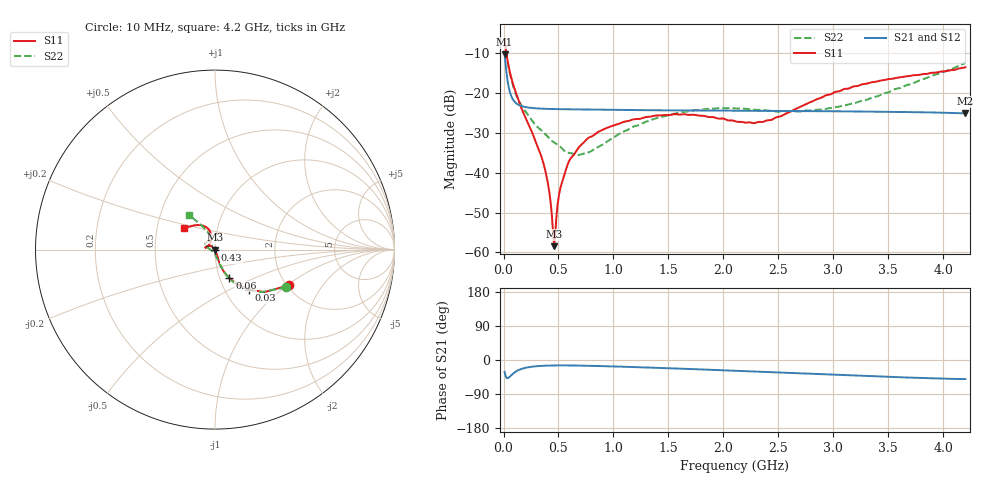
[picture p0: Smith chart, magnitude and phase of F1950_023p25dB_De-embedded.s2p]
! Integrated Device Technology
! Corporate Headquarters
! 6024 Silver Creek Valley Road
! San Jose, CA 95138  USA
! Phone:  1-408-284-8200
! Toll Free:  1-800-223-1366
! Webpage:  http://www.idt.com/
! Timing and RF Division
! 515 Groton Road, Suite 102
! Westford, MA 01886-6024
! Device:  F1950
! Description: 7-bit 0.25 dB Digital Step Attenuator
! Frequency:  150.0 -  4000.00 MHz
! Package:  4x4 mm Thin QFN Plastic Package: 24 pin
! Ports:  2 RF, 12 DC
!  Pin  1  = D0
!  Pin  2  = VDD
!  Pin  3  = Vmode
!  Pin  4  = GND
!  Pin  5  = RF1  =  Port 1
!  Pin  6  = GND
!  Pin  7  = GND
!  Pin  8  = GND
!  Pin  9  = GND
!  Pin 10  = GND
!  Pin 11  = GND
!  Pin 12  = GND
!  Pin 13  = GND
!  Pin 14  = RF2  =  Port 2
!  Pin 15  = GND
!  Pin 16  = LE
!  Pin 17  = CLK
!  Pin 18  = DATE
!  Pin 19  = D6
!  Pin 20  = D5
!  Pin 21  = D4
!  Pin 22  = D3
!  Pin 23  = D2
!  Pin 24  = D1
! State:  93
! Atten State:  23.25 dB
! Voltage:  +5.00 Volts
! Current:  Not Measured mA
! Data:  The device was measured on a the F195X evaluation board which has
!  individual transmission lines to the RF pins.  Data was collected
!  using a calibrated network analyzer.  The evaluation board was
!  de-embedded using a TRL calibration technique.
!  The reference plane is the edge of the package pin.
! Misc:  Board 2019
!  Action Tracker AT0250
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# GHz S dB R 50
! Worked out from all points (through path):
!   420 points, 10 MHz to 4.2 GHz, reference 50 ohm
!   highest |S21| = -10.24 dB at 10 MHz (marker M1); lowest = -25.1 dB at 4.2 GHz (marker M2)
!   group delay of S21, straight-line fit = 23.8 ps
!   lowest |S11| = -58.5 dB at 460 MHz (marker M3), VSWR 1.00, Z = 49.9 - j0.0633 ohm
!   |S11| at or under -10 dB: 26.59 MHz to end of sweep
!   |S22| runs from -35.6 to -6.9 dB; largest |S21 - S12| = 0.00012
!   S11 on the Smith chart (normalised r, x): 10 MHz: 2.06, -1.03; 30 MHz: 1.30, -0.63; 60 MHz: 1.11, -0.36; 430 MHz: 1.00, -0.01; 4.2 GHz: 0.69, +0.17
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0.01  -6.78 -25.7  -10.24 -31.1  -10.24 -31.1  -6.95 -28.0
0.03  -10.63 -49.5  -15.53 -47.8  -15.53 -47.8  -11.02 -51.6
0.06  -15.02 -62.9  -19.94 -43.2  -19.94 -43.2  -15.26 -64.2
0.1  -18.89 -69.8  -22.15 -33.0  -22.15 -33.0  -19.29 -69.4
0.15  -22.83 -71.8  -23.12 -25.0  -23.12 -25.1  -22.50 -73.5
0.35  -36.42 -68.3  -23.92 -15.4  -23.92 -15.4  -29.47 -83.5
0.4  -42.14 -71.3  -23.97 -14.8  -23.97 -14.8  -30.85 -85.3
0.43  -47.86 -81.4  -24.00 -14.5  -23.99 -14.6  -31.71 -88.2
0.45  -54.86 -103.2  -24.01 -14.4  -24.01 -14.4  -32.22 -91.5
0.46  -58.46 -147.9  -24.02 -14.4  -24.02 -14.4  -32.41 -93.1
0.48  -51.46 146.7  -24.03 -14.3  -24.03 -14.3  -32.73 -96.1
0.51  -44.77 137.7  -24.05 -14.3  -24.05 -14.3  -33.28 -99.0
0.57  -39.05 133.1  -24.07 -14.3  -24.07 -14.3  -34.86 -109.6
0.71  -32.93 137.0  -24.13 -14.8  -24.13 -14.9  -35.33 -138.9
1  -28.11 147.3  -24.22 -17.0  -24.22 -17.0  -31.15 178.5
1.41  -25.64 162.6  -24.33 -20.9  -24.32 -20.9  -26.16 160.0
1.73  -25.45 167.9  -24.37 -24.1  -24.37 -24.1  -24.32 151.7
2.11  -27.11 157.3  -24.44 -28.5  -24.44 -28.5  -23.88 141.8
2.43  -26.78 125.5  -24.48 -31.9  -24.48 -32.0  -24.44 130.9
2.81  -22.07 104.8  -24.54 -36.5  -24.54 -36.6  -24.40 115.4
3.51  -16.46 117.0  -24.69 -44.5  -24.69 -44.6  -19.71 112.6
4.2  -13.52 145.5  -25.10 -50.4  -25.09 -50.5  -12.45 126.7
